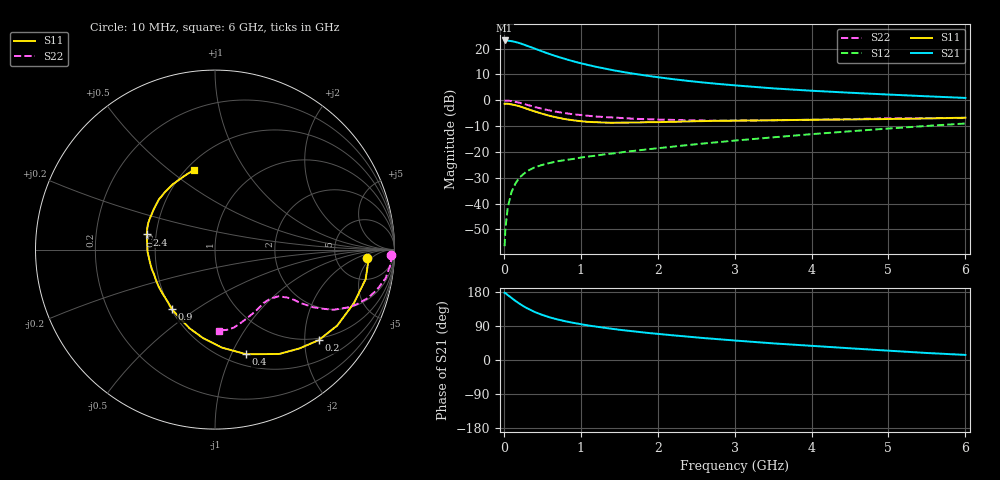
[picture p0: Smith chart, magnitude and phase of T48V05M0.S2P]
! Infineon Technologies  Discrete & RF Semiconductors
! BFR182T
! Si NPN RF Bipolar Junction Transistor in SC75
! VCE = 8 V  IC = 5 mA
! Common Emitter S-Parameters:  October  1999
# GHz  S  MA  R  50
!  f  S11  S21  S12  S22
! GHz  MAG  ANG  MAG  ANG  MAG  ANG  MAG  ANG
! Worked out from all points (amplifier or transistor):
!   36 points, 10 MHz to 6 GHz, reference 50 ohm
!   highest |S21| = 23.1 dB at 10 MHz (marker M1)
!   |S21| within 3 dB of that: start of sweep to 388.7 MHz
!   unconditionally stable (mu >= 1): 1.487 GHz to 4.151 GHz
!   at 250 MHz: K = 0.27, MSG = 25.2 dB, |S12| = -28.7 dB
!   at 1.4 GHz: K = 0.98, MSG = 16.2 dB, |S12| = -20.7 dB
!   at 6 GHz: K = 0.85, MSG = 4.9 dB, |S12| = -9.0 dB
!   lowest NFmin = 1.20 dB at 450 MHz
!   S11 on the Smith chart (normalised r, x): 10 MHz: 11, -4; 200 MHz: 0.95, -2.33; 400 MHz: 0.62, -1.14; 900 MHz: 0.51, -0.40; 2.4 GHz: 0.44, +0.09; 6 GHz: 0.55, +0.61
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0.01  0.8483 -3.3  14.34 177.2  0.0015 71.8  0.9823 -1.7
0.02  0.8585 -3.0  14.34 176.6  0.0032 81.2  0.9832 -1.8
0.05  0.8553 -11.1  14.27 171.5  0.0083 88.9  0.9816 -4.9
0.1  0.8292 -21.1  13.9 163.9  0.0168 80.9  0.9635 -9.6
0.15  0.802 -31.8  13.41 156.1  0.0243 73.3  0.9309 -13.8
0.2  0.7667 -41.2  12.81 149.1  0.0314 71.1  0.8955 -17.4
0.25  0.7237 -49.6  12.07 142.7  0.0367 66.0  0.8536 -20.6
0.3  0.6827 -58.4  11.35 136.8  0.0422 63.4  0.8166 -23.1
0.4  0.6082 -73.4  10.01 126.8  0.0502 58.4  0.7411 -26.9
0.5  0.5473 -86.0  8.794 119.0  0.0561 55.4  0.6813 -28.9
0.6  0.4974 -97.7  7.781 112.3  0.0613 54.0  0.6321 -30.5
0.7  0.4608 -107.9  6.957 106.9  0.066 53.3  0.5922 -31.3
0.9  0.4095 -125.7  5.682 98.2  0.073 53.0  0.5355 -32.3
1.1  0.381 -140.3  4.79 91.0  0.0815 53.6  0.4998 -33.1
1.3  0.3701 -152.8  4.143 85.2  0.0894 54.7  0.4735 -34.1
1.6  0.3692 -167.7  3.418 77.5  0.1015 56.1  0.4463 -35.7
2.2  0.3822 172.6  2.557 65.1  0.1267 58.8  0.4165 -40.9
2.4  0.3893 167.5  2.361 61.5  0.1361 59.6  0.4089 -43.1
3.5  0.4093 146.0  1.697 43.9  0.1915 60.1  0.4103 -56.2
4.5  0.4247 131.2  1.397 30.9  0.2507 57.9  0.4313 -69.9
5.5  0.4435 113.2  1.192 18.5  0.3184 53.9  0.452 -82.1
6  0.4597 104.8  1.108 13.4  0.3549 50.8  0.4516 -87.3
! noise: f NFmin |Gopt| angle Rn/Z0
0.45  1.2  0.27  37  0.3
0.9  1.3  0.25  75  0.23
1.8  1.9  0.21  145  0.2
